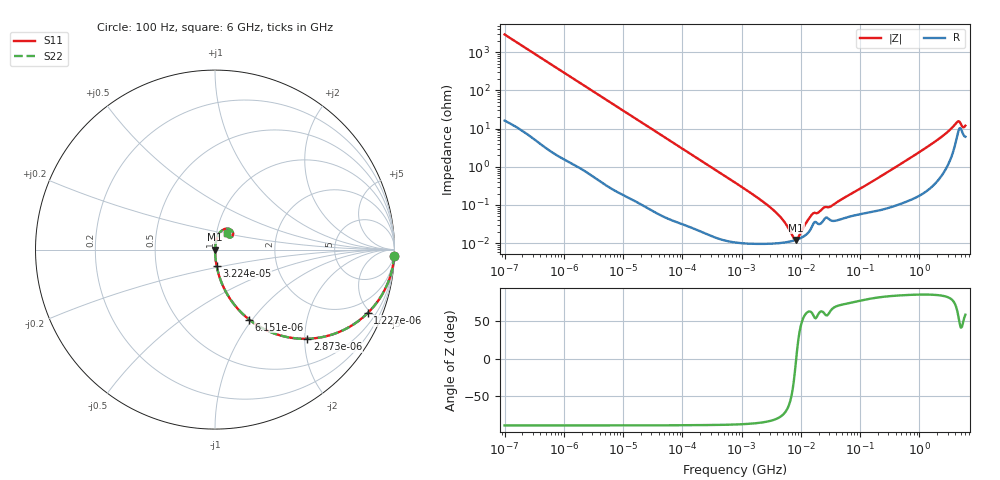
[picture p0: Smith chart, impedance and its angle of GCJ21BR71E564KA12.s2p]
!Murata Part Number: GCJ21BR71E564KA12
!These Parameters are Measured in Series Mode Connection
!Data Generated on Mar 13, 2026
!  o--ll--o
!Port1  Port2
!  o------o
!Operation Temp=25[degC], DC Bias Voltage=0[V]
!Freq. Start=100[Hz] Stop=6[GHz] 401[Steps]
# Hz S RI R 50
!Freq.(Hz) S11(Real) S11(Imag) S21(Real) S21(Imag) S12(Real) S12(Imag) S22(Real) S22(Imag)
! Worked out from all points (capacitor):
!   401 points, 100 Hz to 6 GHz, reference 50 ohm
!   read as one part in series: C = 544 nF near 109 Hz
!   lowest |Z| = 12.2 mohm at 8.312 MHz (marker M1)
!   series resonance near 8.365 MHz, so ESL is about 670 pH
!   S11 on the Smith chart (normalised r, x): 100 Hz: 1, -58; 1.227 kHz: 1.03, -4.80; 2.873 kHz: 1.01, -2.06; 6.151 kHz: 1.01, -0.96; 32.24 kHz: 1.00, -0.19; 6 GHz: 1.12, +0.20
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100  0.9986 -0.0342  0.00136 0.0342  0.00136 0.0342  0.9986 -0.0342
401  0.9811 -0.1337  0.0189 0.1337  0.0189 0.1337  0.9811 -0.1337
1227  0.8509 -0.3534  0.1491 0.3534  0.1491 0.3534  0.8509 -0.3534
2008  0.6829 -0.4624  0.3171 0.4624  0.3171 0.4624  0.6829 -0.4624
2873  0.5145 -0.4969  0.4855 0.4969  0.4855 0.4969  0.5145 -0.4969
6151  0.19 -0.3895  0.81 0.3895  0.81 0.3895  0.19 -0.3895
12041  0.0588 -0.232  0.9412 0.232  0.9412 0.232  0.0588 -0.232
32244  0.00916 -0.0917  0.9908 0.0917  0.9908 0.0917  0.00916 -0.0917
40335  0.00601 -0.0736  0.994 0.0736  0.994 0.0736  0.00601 -0.0736
774597  0.000119 -0.00387  0.9999 0.00387  0.9999 0.00387  0.000119 -0.00387
3549919  9.85e-05 -0.0007  0.9999 0.0007  0.9999 0.0007  9.85e-05 -0.0007
5079039  0.000103 -0.000378  0.9999 0.000378  0.9999 0.000378  0.000103 -0.000378
7599586  0.000117 -7e-05  0.9999 7e-05  0.9999 7e-05  0.000117 -7e-05
8311524  0.000122 -4.6e-06  0.9999 4.6e-06  0.9999 4.6e-06  0.000122 -4.6e-06
9090158  0.000128 6.13e-05  0.9999 -6.13e-05  0.9999 -6.13e-05  0.000128 6.13e-05
1.243624e7  0.00017 0.000307  0.9998 -0.000307  0.9998 -0.000307  0.00017 0.000307
1.555665e7  0.000278 0.0005  0.9997 -0.0005  0.9997 -0.0005  0.000278 0.0005
3.330331e7  0.000387 0.000872  0.9996 -0.000872  0.9996 -0.000872  0.000387 0.000872
3.124326e8  0.00091 0.00771  0.9991 -0.00771  0.9991 -0.00771  0.00091 0.00771
1.873145e9  0.00581 0.046  0.9942 -0.046  0.9942 -0.046  0.00581 0.046
4.193612e9  0.0617 0.117  0.9383 -0.117  0.9383 -0.117  0.0617 0.117
6e9  0.0665 0.0898  0.9335 -0.0898  0.9335 -0.0898  0.0665 0.0898
